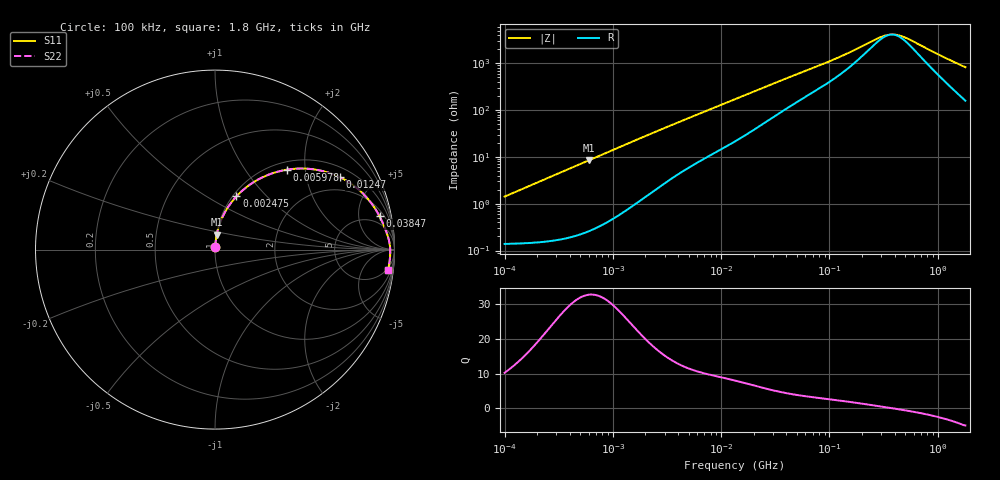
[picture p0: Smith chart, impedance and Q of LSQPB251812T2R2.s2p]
! LSQPB251812T2R2  S-PARAMETER MODEL  ( General Type )
! Model Generated by TAIYO YUDEN Corporation (http://www.ty-top.com)
! Version 3.0
! TAIYO YUDEN Control No. 110926NF18SB-HKC
! Copyright(c) 2007 TAIYO YUDEN CO.,LTD. All Rights Reserved.
! Product Description (link to TY-COMPAS)
! https://ds.yuden.co.jp/TYCOMPAS/or/detail?pn=LSQPB251812T2R2M&u=M
! Products Name : Inductors
! Characteristics :
!  Inductance : 2.2 uH , SRF(min) : 80 MHz , DC Resistance(max) : 0.1755 Ohm
!  Rated Current : Saturation :1000 mA , Temp Rise : 850 mA (40 degC)
!  Case Size : 2.5 x 1.8 / 0.098 x 0.071 [mm/inch] , Thickness : 1.2 / 0.048 [mm/inch]
!  (Conditions: Temperature = 25 degC , DC Bias Current/Voltage = 0A / 0V)
! External Node Assignments :
!  1  o---GGG---o  2
! GND o---------o GND
! Frequency Range : 0.1MHz  -  1800MHz  [ 402 STEP ]
# MHz S RI R 50
! Freq[MHz].  S11 Real  S11 Imag  S21 Real  S21 Imag  S12 Real  S12 Imag  S22 Real  S22 Imag
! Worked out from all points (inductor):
!   401 points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, 100 kHz to 1.8 GHz, reference 50 ohm
!   read as one part in series: L = 2.25 uH near 105 kHz
!   highest Q = 32.8 at 597.8 kHz (marker M1), where L = 2.25 uH
!   self-resonance near 375.4 MHz
!   S11 on the Smith chart (normalised r, x): 100 kHz: 1.00, +0.03; 2.475 MHz: 1.04, +0.69; 5.978 MHz: 1.15, +1.59; 12.47 MHz: 1.39, +3.18; 38.47 MHz: 3.02, +8.96; 1.8 GHz: 4, -16
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0.1  0.00158 0.0141  0.9984 -0.0141  0.9984 -0.0141  0.00158 0.0141
0.253659  0.00285 0.0357  0.9972 -0.0357  0.9972 -0.0357  0.00285 0.0357
0.516129  0.00751 0.0722  0.9925 -0.0722  0.9925 -0.0722  0.00751 0.0722
0.597843  0.00959 0.0834  0.9904 -0.0834  0.9904 -0.0834  0.00959 0.0834
1.374945  0.0428 0.1835  0.9572 -0.1835  0.9572 -0.1835  0.0428 0.1835
2.475151  0.1196 0.2968  0.8804 -0.2968  0.8804 -0.2968  0.1196 0.2968
2.66389  0.1348 0.3124  0.8652 -0.3124  0.8652 -0.3124  0.1348 0.3124
3.942096  0.2417 0.3911  0.7583 -0.3911  0.7583 -0.3911  0.2417 0.3911
5.97828  0.399 0.4449  0.601 -0.4449  0.601 -0.4449  0.399 0.4449
8.632747  0.5549 0.4464  0.4451 -0.4464  0.4451 -0.4464  0.5549 0.4464
12.46584  0.6977 0.4024  0.3023 -0.4024  0.3023 -0.4024  0.6977 0.4024
13.41641  0.7224 0.3894  0.2776 -0.3894  0.2776 -0.3894  0.7224 0.3894
21.89777  0.8462 0.2893  0.1538 -0.2893  0.1538 -0.2893  0.8462 0.2893
38.46609  0.9166 0.1857  0.0834 -0.1857  0.0834 -0.1857  0.9166 0.1857
69.24595  0.9498 0.1118  0.0502 -0.1118  0.0502 -0.1118  0.9498 0.1118
134.1607  0.9679 0.057  0.0321 -0.057  0.0321 -0.057  0.9679 0.057
286.6876  0.9755 0.0133  0.0245 -0.0133  0.0245 -0.0133  0.9755 0.0133
357.3983  0.9762 0.00241  0.0238 -0.00241  0.0238 -0.00241  0.9762 0.00241
424.248  0.9765 -0.00603  0.0235 0.00603  0.0235 0.00603  0.9765 -0.00603
503.6016  0.9765 -0.0147  0.0235 0.0147  0.0235 0.0147  0.9765 -0.0147
1102.831  0.9729 -0.064  0.0271 0.064  0.0271 0.064  0.9729 -0.064
1800  0.9642 -0.1121  0.0358 0.1121  0.0358 0.1121  0.9642 -0.1121
